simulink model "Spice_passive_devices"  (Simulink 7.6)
settings: Solver=ode15s  StartTime=0.0  StopTime=0.03  RelTol=1e-3
StopFcn:
  | clc, close all
  | load Upont_Icommande.mat
  | plotyy(x(1,:),x(2,:), x(1,:),x(3,:))
  | grid
  | title('U_pont diviseur et Courant de commande du switch')
  | xlabel('temps')
libraries: fl_lib x9, elec_lib x4, nesl_utility x4

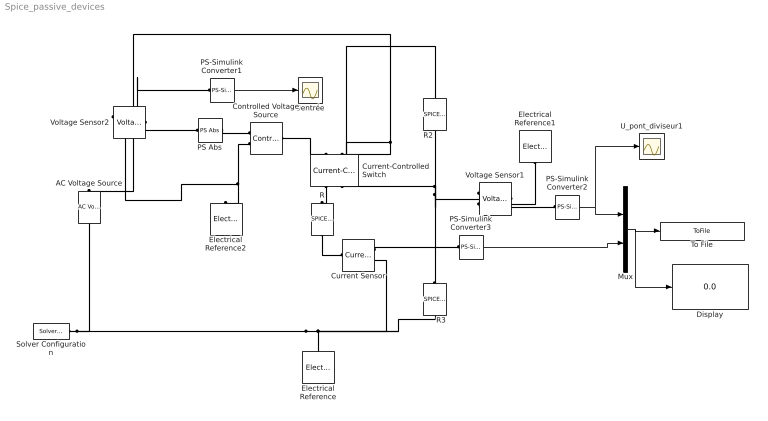
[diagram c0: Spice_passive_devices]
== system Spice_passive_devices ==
  AC Voltage Source : fl_lib/Electrical/Electrical Sources/AC Voltage Source  DialogController=NetworkEngine.DynNeDlgSource  SystemSampleTime=-1  amp=150 V  shift=0 rad  omega=60 Hz  i_Log=off  v_Log=off  LocalVarNames=|i|v  LocalVarDescs=|i|v  LocalVarLogging=[0 0]
  Controlled Voltage Source : fl_lib/Electrical/Electrical Sources/Controlled Voltage Source  DialogController=NetworkEngine.DynNeDlgSource  SystemSampleTime=-1  i_Log=off  v_Log=off  LocalVarNames=|i|v  LocalVarDescs=|i|v  LocalVarLogging=[0 0]
  Current Sensor : fl_lib/Electrical/Electrical Sensors/Current Sensor  DialogController=NetworkEngine.DynNeDlgSource  SystemSampleTime=-1  i1_Log=off  v1_Log=off  LocalVarNames=|i1|v1  LocalVarDescs=|i1|v1  LocalVarLogging=[0 0]
  Current-Controlled Switch : elec_lib/Additional Components/SPICE-Compatible Components/Passive Devices/Current-Controlled Switch  DialogController=NetworkEngine.DynNeDlgSource  SystemSampleTime=-1  IT=10 A  IH=3 A  RON=1 Ohm  ROFF=1e+12 Ohm  IC_state=-1  LocalVarLogging=[]
  Display : Display
  Electrical Reference : fl_lib/Electrical/Electrical Elements/Electrical Reference  DialogController=NetworkEngine.DynNeDlgSource  SystemSampleTime=-1  i_Log=off  LocalVarNames=|i  LocalVarDescs=|i  LocalVarLogging=0
  Electrical Reference1 : fl_lib/Electrical/Electrical Elements/Electrical Reference  DialogController=NetworkEngine.DynNeDlgSource  SystemSampleTime=-1  i_Log=off  LocalVarNames=|i  LocalVarDescs=|i  LocalVarLogging=0
  Electrical Reference2 : fl_lib/Electrical/Electrical Elements/Electrical Reference  DialogController=NetworkEngine.DynNeDlgSource  SystemSampleTime=-1  i_Log=off  LocalVarNames=|i  LocalVarDescs=|i  LocalVarLogging=0
  Mux : Mux  Inputs=2
  PS Abs : fl_lib/Physical Signals/Nonlinear Operators/PS Abs  DialogController=NetworkEngine.DynNeDlgSource  SystemSampleTime=-1  LocalVarLogging=[]
  PS-Simulink Converter1 : nesl_utility/PS-Simulink Converter  DialogController=NetworkEngine.DynNeUtilDlgSource  SystemSampleTime=-1  PhysicalDomain=network_engine_domain  LeftPortType=input  RightPortType=output  SubClassName=ps_output  Unit=1  AffineConversion=off
  PS-Simulink Converter2 : nesl_utility/PS-Simulink Converter  DialogController=NetworkEngine.DynNeUtilDlgSource  SystemSampleTime=-1  PhysicalDomain=network_engine_domain  LeftPortType=input  RightPortType=output  SubClassName=ps_output  Unit=1  AffineConversion=off
  PS-Simulink Converter3 : nesl_utility/PS-Simulink Converter  DialogController=NetworkEngine.DynNeUtilDlgSource  SystemSampleTime=-1  PhysicalDomain=network_engine_domain  LeftPortType=input  RightPortType=output  SubClassName=ps_output  Unit=1  AffineConversion=off
  R : elec_lib/Additional Components/SPICE-Compatible Components/Passive Devices/SPICE Resistor  DialogController=NetworkEngine.DynNeDlgSource  SystemSampleTime=-1  SCALE=1  R_param=1  R=10 Ohm  RSH=0 Ohm  LENGTH=1e-6 m  WIDTH=1e-6 m  NARROW=0 m  T_param=1  TC1=0 1/K  TC2=0 1/K^2  TOFFSET=0 K  TFIXED=300.15 K  TMEAS=300.15 K  LocalVarLogging=[]
  R2 : elec_lib/Additional Components/SPICE-Compatible Components/Passive Devices/SPICE Resistor  DialogController=NetworkEngine.DynNeDlgSource  SystemSampleTime=-1  SCALE=1  R_param=1  R=10 Ohm  RSH=0 Ohm  LENGTH=1e-6 m  WIDTH=1e-6 m  NARROW=0 m  T_param=1  TC1=0 1/K  TC2=0 1/K^2  TOFFSET=0 K  TFIXED=300.15 K  TMEAS=300.15 K  LocalVarLogging=[]
  R3 : elec_lib/Additional Components/SPICE-Compatible Components/Passive Devices/SPICE Resistor  DialogController=NetworkEngine.DynNeDlgSource  SystemSampleTime=-1  SCALE=1  R_param=1  R=5 Ohm  RSH=0 Ohm  LENGTH=1e-6 m  WIDTH=1e-6 m  NARROW=0 m  T_param=1  TC1=0 1/K  TC2=0 1/K^2  TOFFSET=0 K  TFIXED=300.15 K  TMEAS=300.15 K  LocalVarLogging=[]
  Solver Configuration : nesl_utility/Solver Configuration  DialogController=NetworkEngine.DynNeUtilDlgSource  SystemSampleTime=-1  PhysicalDomain=network_engine_domain  LeftPortType=input  RightPortType=generic  SubClassName=solver  Accelerate=off  Profile=off  ResidualTolerance=1e-9  MaxNonlinIter=12  MaxModeIter=2  DoFixedCost=off  UseLocalSampling=off  DoDC=off  LinearAlgebra=Sparse  LocalSolverSampleTime=.001  LocalSolverChoice=NE_BACKWARD_EULER_ADVANCER  UseLocalSolver=off
  To File : ToFile  Filename=Upont_Icommande  MatrixName=x
  U_pont_diviseur1 : Scope
  Uentrée : Scope
  Voltage Sensor1 : fl_lib/Electrical/Electrical Sensors/Voltage Sensor  DialogController=NetworkEngine.DynNeDlgSource  SystemSampleTime=-1  i1_Log=off  v1_Log=off  LocalVarNames=|i1|v1  LocalVarDescs=|i1|v1  LocalVarLogging=[0 0]
  Voltage Sensor2 : fl_lib/Electrical/Electrical Sensors/Voltage Sensor  DialogController=NetworkEngine.DynNeDlgSource  SystemSampleTime=-1  i1_Log=off  v1_Log=off  LocalVarNames=|i1|v1  LocalVarDescs=|i1|v1  LocalVarLogging=[0 0]
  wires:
  PS-Simulink Converter2/1 -> Mux/1, U_pont_diviseur1/1
  Mux/1 -> To File/1, Display/1
  PS-Simulink Converter1/1 -> Uentrée/1
  PS-Simulink Converter3/1 -> Mux/2
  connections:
  R2/RConn1 -- Voltage Sensor1/LConn1 -- Current-Controlled Switch/RConn2 -- R3/LConn1
  Current-Controlled Switch/RConn1 -- R/LConn1
  R/RConn1 -- Current Sensor/LConn1
  Current Sensor/RConn1 -- PS-Simulink Converter3/LConn1
  Voltage Sensor1/RConn1 -- PS-Simulink Converter2/LConn1
  Electrical Reference1/LConn1 -- Voltage Sensor1/RConn2
  Voltage Sensor2/LConn1 -- R2/LConn1 -- Current-Controlled Switch/LConn2 -- AC Voltage Source/LConn1
  Solver Configuration/RConn1 -- Electrical Reference/LConn1 -- R3/RConn1 -- Current Sensor/RConn2 -- AC Voltage Source/RConn1
  Controlled Voltage Source/LConn1 -- Current-Controlled Switch/LConn1
  Voltage Sensor2/RConn1 -- PS Abs/LConn1 -- PS-Simulink Converter1/LConn1
  PS Abs/RConn1 -- Controlled Voltage Source/RConn1
  Controlled Voltage Source/RConn2 -- Electrical Reference2/LConn1 -- Voltage Sensor2/RConn2
